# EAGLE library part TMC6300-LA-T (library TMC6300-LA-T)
Highly Efficient Low Voltage, Zero Standby Current Driver for 3-Phase BLDC/PMSM Motors up to 2A peak, Triple Half-Bridge with separate HS and LS control signals Source: Datasheet
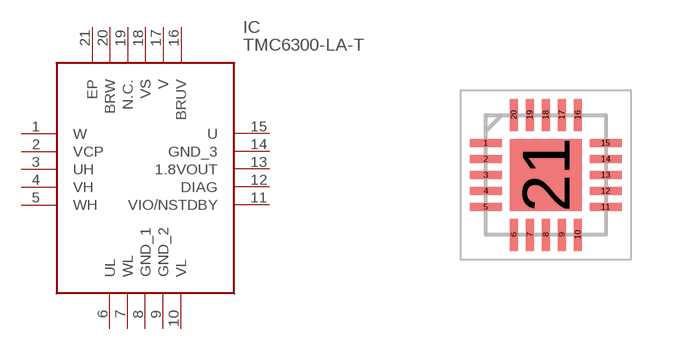
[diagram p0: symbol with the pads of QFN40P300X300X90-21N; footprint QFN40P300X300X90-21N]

Designator prefix IC

## TMC6300-LA-T (Description: Highly Efficient Low Voltage, Zero Standby Current Driver for 3-Phase BLDC/PMSM Motors up to 2A peak, Triple Half-Bridge with separate HS and LS control signals; Height: 0.9mm; Manufacturer_Name: Analog Devices; Manufacturer_Part_Number: TMC6300-LA-T; Mouser_Part_Number: 700-TMC6300-LA-T; Mouser_Price-Stock: https://www.mouser.co.uk/ProductDetail/ADI-Trinamic/TMC6300-LA-T?qs=TiOZkKH1s2SPDan6zA6fKg%3D%3D)  [QFN40P300X300X90-21N]
1  W
2  VCP
3  UH
4  VH
5  WH
6  UL
7  WL
8  GND_1
9  GND_2
10  VL
11  VIO/NSTDBY
12  DIAG
13  1.8VOUT
14  GND_3
15  U
16  BRUV
17  V
18  VS
19  N.C.  nc
20  BRW
21  EP

## Footprint QFN40P300X300X90-21N (pad centres in mm)
QFN20_2023
smd 0.8 x 0.2: 1 -1.5,0.8; 2 -1.5,0.4; 3 -1.5,0; 4 -1.5,-0.4; 5 -1.5,-0.8; 11 1.5,-0.8; 12 1.5,-0.4; 13 1.5,0; 14 1.5,0.4; 15 1.5,0.8
smd 0.2 x 0.8: 6 -0.8,-1.5; 7 -0.4,-1.5; 8 0,-1.5; 9 0.4,-1.5; 10 0.8,-1.5; 16 0.8,1.5; 17 0.4,1.5; 18 0,1.5; 19 -0.4,1.5; 20 -0.8,1.5
smd 1.8 x 1.8: 21 0,0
